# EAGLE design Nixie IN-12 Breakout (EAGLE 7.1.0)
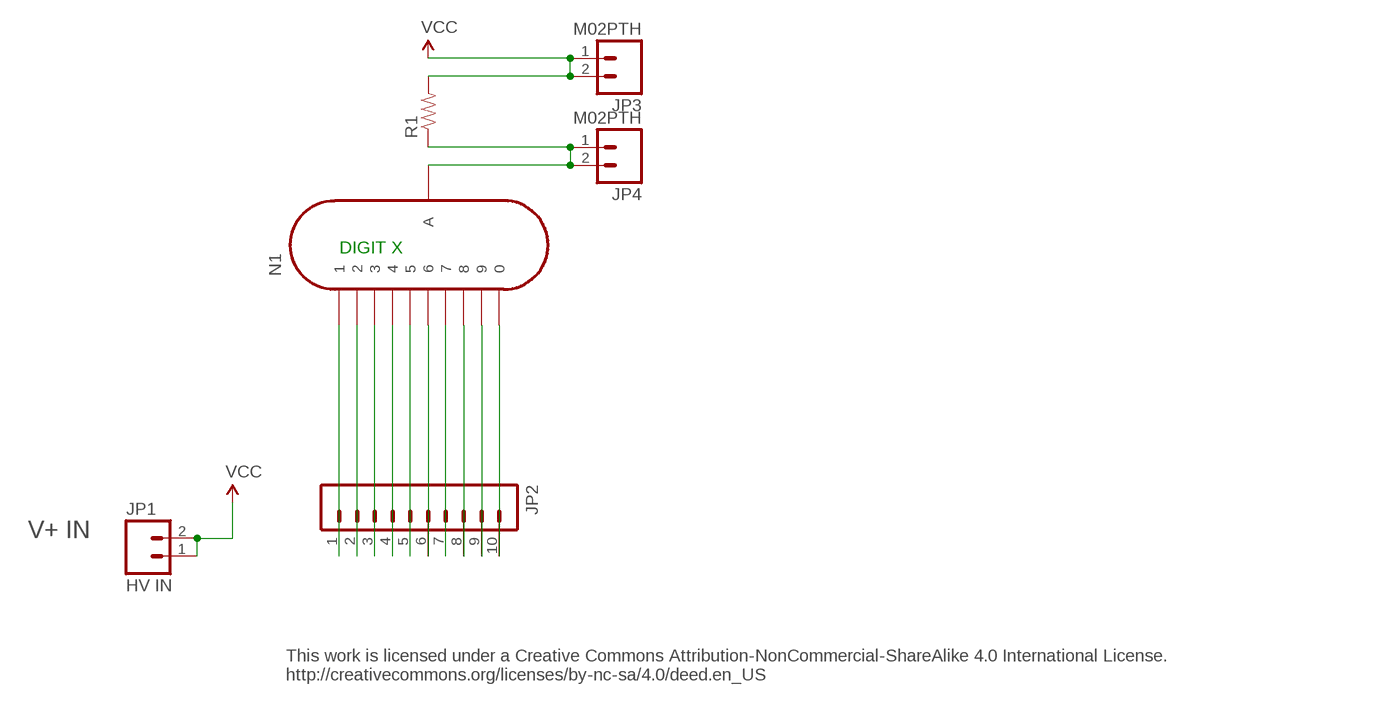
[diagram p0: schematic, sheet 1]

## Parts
JP1  HV IN  M02PTH  [1X02]
JP2  M10"  [1X10]
JP3  M02PTH  [1X02]
JP4  M02PTH  [1X02]
N1  IN-12A  [IN-12]
R1  RESISTORPTH-1/4W  [AXIAL-0.4]

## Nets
N$1: JP2.6 N1.6
N$2: JP2.9 N1.9
N$3: JP2.8 N1.8
N$4: JP2.10 N1.0
N$5: JP2.7 N1.7
N$6: JP2.5 N1.5
N$7: JP2.4 N1.4
N$8: JP2.3 N1.3
N$9: JP2.2 N1.2
N$10: JP2.1 N1.1
N$19: JP4.1 JP4.2 N1.A R1.P$1
VCC: JP1.1 JP1.2 JP3.1 JP3.2 R1.P$2

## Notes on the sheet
- DIGIT X
- V+ IN
- This work is licensed under a Creative Commons Attribution-NonCommercial-ShareAlike 4.0 International License.
  http://creativecommons.org/licenses/by-nc-sa/4.0/deed.en_US

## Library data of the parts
JP1 JP3 JP4 = SparkFun-Connectors:M02: Standard 2-pin 0.1" header. Use with
JP2 = SparkFun-Connectors:M10: Header 10 Standard 10-pin 0.1" header. Use with straight break away headers (SKU : PRT-00116), right angle break away headers (PRT-00553), swiss pins (PRT-00743), machine pins (PRT-00117), and female headers (PRT-00115).
N1 = Nixie Tubes 2:IN-12A: IN-12A: medium numeric topview nixie tube
R1 = SparkFun-Resistors:RESISTOR: Resistor

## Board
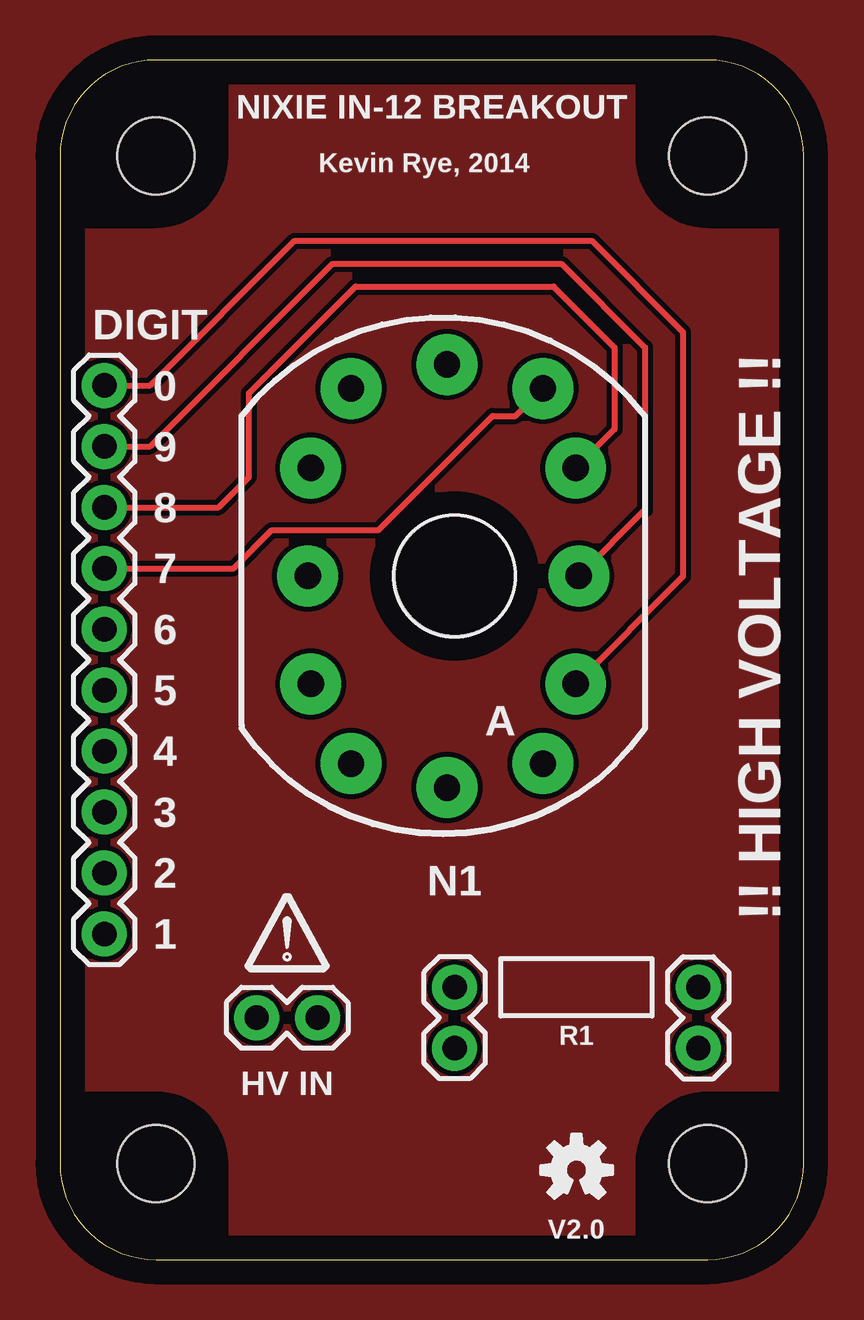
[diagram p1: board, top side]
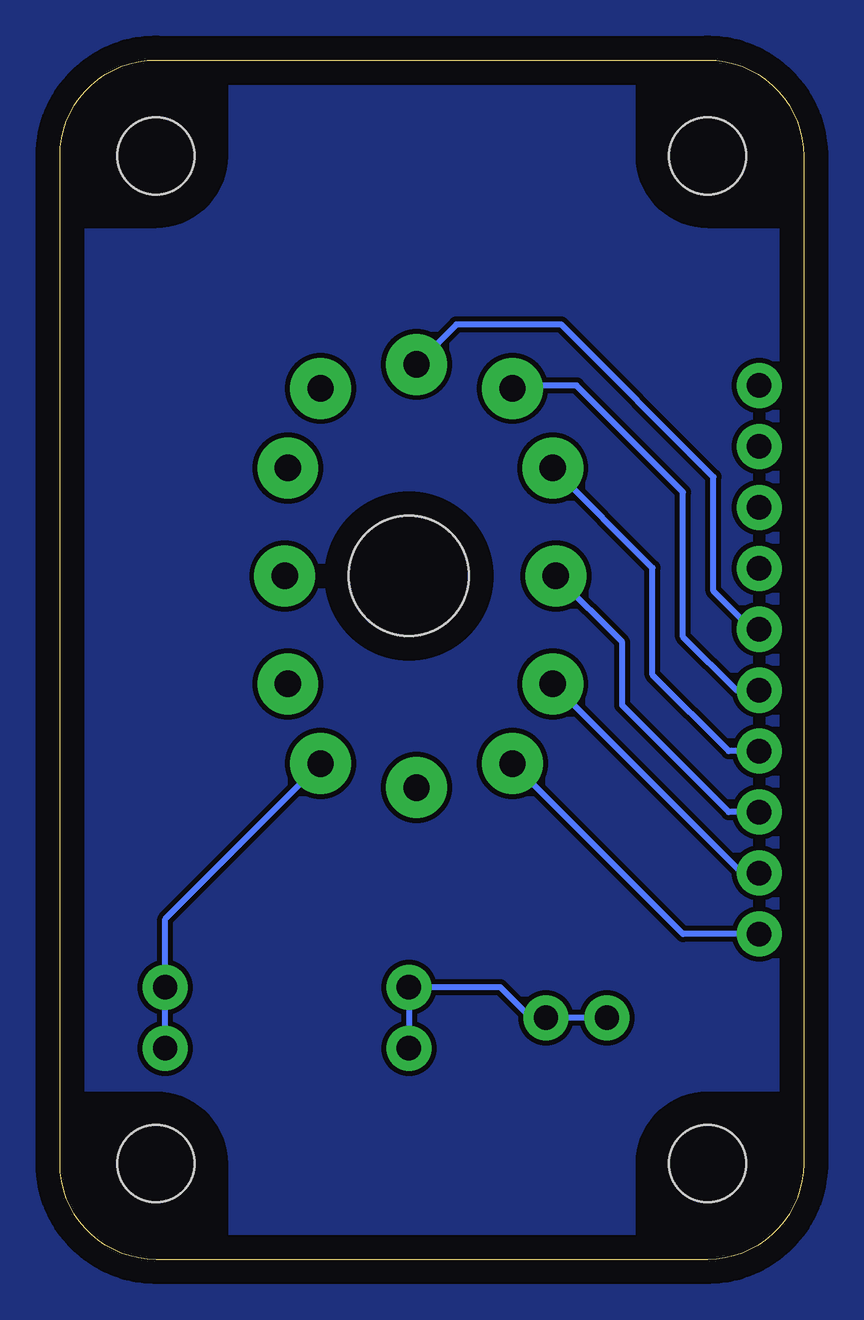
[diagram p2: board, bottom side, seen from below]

Size 31 x 50 mm. Coordinates in mm from the lower left corner, seen from the top.
Copper layers (1*16): Top 0.035mm / dielectric 1.5mm / Bottom 0.035mm
Design rules "default": minimum track width 10mil, minimum drill 24mil, track to track 8mil, track to pad 8mil, pad to pad 8mil, via to via 8mil, smd to smd 8mil, copper to edge 40mil, drill to drill 8mil, minimum pad ring 10mil, minimum via ring 8mil, stop-mask expansion 4mil, vias tented up to drill 0mil, thermal gap 10mil

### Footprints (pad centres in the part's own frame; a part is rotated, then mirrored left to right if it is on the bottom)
1X02 = drill 1.016 pad 1.88: 1 0,0; 2 2.54,0
1X10 = drill 1.016 pad 1.88: 1 0,0; 2 2.54,0; 3 5.08,0; 4 7.62,0; 5 10.16,0; 6 12.7,0; 7 15.24,0; 8 17.78,0; 9 20.32,0; 10 22.86,0
IN-12 = drill 1.1 pad 2.54: 0 5.048,-4.5; 1 -4.317,-7.817; 2 -6,-4.5; 3 -6.127,0; 4 -6,4.5; 5 -4.317,7.817; 6 -0.318,8.818; 7 3.683,7.817; 8 5.048,4.5; 9 5.175,0; A 3.683,-7.817; LHDP -0.318,-8.818 | hole 5: 0,0
AXIAL-0.4 = drill 0.9 pad 1.88: P$1 -5.08,0; P$2 5.08,0
DP5031_V1 = hole 3.2: -21,-11.5; 21,-11.5; 21,11.5; -21,11.5

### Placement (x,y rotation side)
JP1  8.2,10.08 0 top
JP2  1.85,13.57 90 top
JP3  16.45,11.35 270 top
JP4  26.61,8.81 90 top
N1  16.45,28.49 0 top
R1  21.53,11.35 180 top
U$1  [DP5031_V1]  15.5,25 90 top
U$4  [OSHW-LOGO-S]  21.53,3.73 0 top
U$6  [DP_LOGO]  9.47,12.62 0 top

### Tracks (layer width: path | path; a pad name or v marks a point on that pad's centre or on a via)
GND
  pour Bottom: 39.31,54.84 39.31,-5.16 -5.77,-5.16 -5.77,54.84
  pour Top: -4.18,53.57 37.41,53.57 37.41,-4.21 -4.18,-4.21
N$1
  Bottom 0.254: JP2.6 2.17,26.27 3.75,27.86 3.75,32.62 10.1,38.97 14.48,38.97 N1.6
N$2
  Top 0.254: JP2.9 3.75,33.89 11.37,41.51 20.9,41.51 24.39,38.02 24.39,31.25 N1.9
N$3
  Top 0.254: JP2.8 6.61,31.35 7.88,32.62 7.88,36.11 12.33,40.56 20.58,40.56 23.12,38.02 23.12,34.61 N1.8
N$4
  Top 0.254: JP2.10 3.75,36.43 9.79,42.46 22.17,42.46 25.98,38.65 25.98,28.47 N1.0
N$5
  Top 0.254: JP2.7 7.25,28.81 8.83,30.4 13.28,30.4 18.04,35.16 18.99,35.16 N1.7
N$6
  Bottom 0.254: JP2.5 2.8,23.73 5.02,25.95 5.02,31.98 9.47,36.43 12.02,36.43 N1.5
N$7
  Bottom 0.254: JP2.4 3.12,21.19 6.29,24.36 6.29,28.83 N1.4
N$8
  Bottom 0.254: JP2.3 3.12,18.65 7.56,23.09 7.56,25.73 N1.3
N$9
  Bottom 0.254: JP2.2 2.57,16.11 N1.2
N$10
  Bottom 0.254: JP2.1 5.03,13.57 N1.1
N$19
  Bottom 0.254: JP4.1 JP4.2 26.61,14.2 N1.A
VCC
  Bottom 0.254: JP1.1 JP1.2 11.37,10.08 12.64,11.35 JP3.1 JP3.2

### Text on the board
Unrouted: This work is licensed under a Creative Commons Attribution-NonCommercial-ShareAlike 4.0 International License. / http://creativecommons.org/licenses/by-nc-sa/4.0/deed.en_US
tNames: NIXIE IN-12 BREAKOUT | Kevin Rye, 2014 | DIGIT | 0 | 9 | 8 | 7 | 6 | !! HIGH VOLTAGE !! | 5 | A | 4 | 3 | 2 | 1 | V2.0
